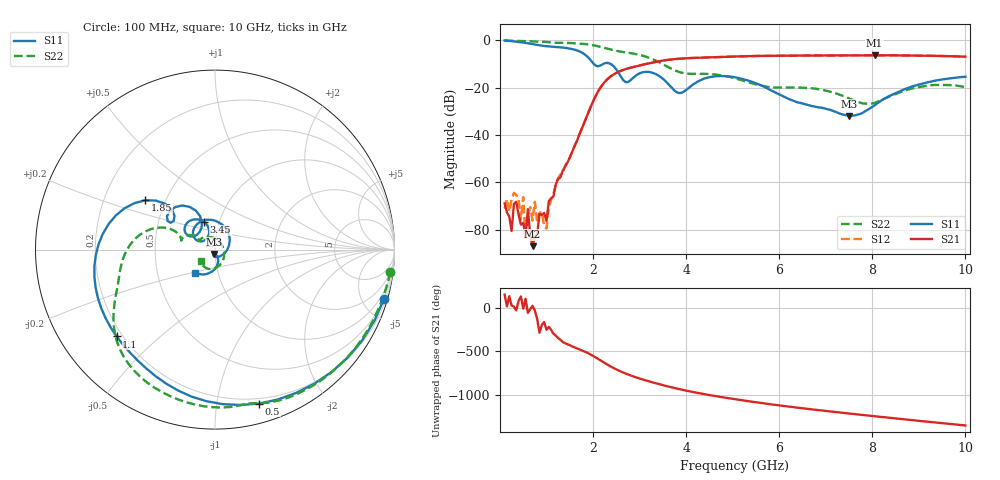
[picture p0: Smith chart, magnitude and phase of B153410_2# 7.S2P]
!  2-Port S-parameters saved by WinCal
! VAR MeasName=S-Parameters (CALIBRATED_DATA) read from VNA (N5245A)
! VAR MeasDate=2016-12-23 9:59:42
! VAR NAME=B153410_2# 7
! VAR FILENAME=B153410_2# 7.S2P
! VAR DATE=2016-12-23 9:59:42
! VAR PHYS_PORTS=1,2
# Hz S DB R 50
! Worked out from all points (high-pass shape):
!   199 points, 100 MHz to 10 GHz, reference 50 ohm
!   highest |S21| = -6.38 dB at 8.05 GHz (marker M1); lowest = -86.9 dB at 700 MHz (marker M2)
!   |S21| within 3 dB of the highest: 3.296 GHz to end of sweep
!   lowest |S11| = -32.0 dB at 7.5 GHz (marker M3), VSWR 1.05, Z = 49.4 - j2.4 ohm
!   |S11| at or under -10 dB: 2.017 GHz to 2.224 GHz (207.2 MHz wide, 9.77 % of centre); 2.372 GHz to end of sweep
!   |S22| runs from -26.8 to -0.1 dB; largest |S21 - S12| = 0.0025
!   S11 on the Smith chart (normalised r, x): 100 MHz: 0.47, -7.01; 500 MHz: 0.16, -1.31; 1.1 GHz: 0.18, -0.37; 1.85 GHz: 0.39, +0.27; 3.45 GHz: 0.84, +0.27; 10 GHz: 0.78, -0.21
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1e8  -0.16 -16.2  -68.89 153.9  -71.07 -163.3  -0.13 -7.4
2.5e8  -0.41 -39.0  -80.52 27.9  -67.11 -176.6  -0.25 -17.6
3e8  -0.52 -46.3  -69.11 14.4  -64.44 -135.8  -0.29 -21.0
4.5e8  -0.86 -67.4  -77.84 132.8  -75.71 71.5  -0.37 -30.9
5e8  -0.99 -74.1  -77.12 -7.9  -66.19 137.3  -0.39 -34.2
5.5e8  -1.14 -80.6  -82.77 104.6  -84.47 -122.6  -0.42 -37.5
6e8  -1.28 -87.0  -71.32 -57.1  -73.78 -102.6  -0.45 -40.8
7e8  -1.63 -99.1  -86.92 23.5  -76.09 133.4  -0.52 -47.4
7.5e8  -1.82 -104.8  -82.94 -29.4  -68.18 33.5  -0.56 -50.7
1e9  -2.56 -129.4  -76.26 108.6  -79.48 -149.3  -0.79 -67.1
1.1e9  -2.72 -138.5  -66.68 109.3  -67.33 104.8  -0.98 -73.4
1.75e9  -5.14 155.3  -37.69 -125.0  -37.78 -124.7  -1.51 -113.5
1.85e9  -6.47 144.7  -32.91 -148.7  -32.91 -149.0  -1.70 -120.3
2.35e9  -9.78 133.1  -15.77 56.3  -15.76 56.4  -3.82 -150.7
3.4e9  -14.87 115.3  -8.98 -152.6  -8.96 -152.7  -9.12 159.8
3.45e9  -15.53 111.9  -8.80 -159.8  -8.79 -159.9  -9.63 158.1
5.05e9  -15.68 93.9  -6.90 31.4  -6.92 31.4  -16.10 148.8
6.7e9  -27.80 -77.8  -6.48 -85.1  -6.49 -85.1  -20.30 138.6
7.5e9  -32.04 -103.5  -6.41 -132.9  -6.41 -132.9  -24.56 84.5
8.05e9  -27.44 -72.6  -6.38 -164.3  -6.38 -164.3  -26.44 1.2
8.35e9  -23.74 -74.2  -6.41 178.8  -6.39 179.0  -23.89 -38.2
1e10  -15.43 -130.0  -6.97 90.0  -6.95 90.1  -19.81 -140.9
